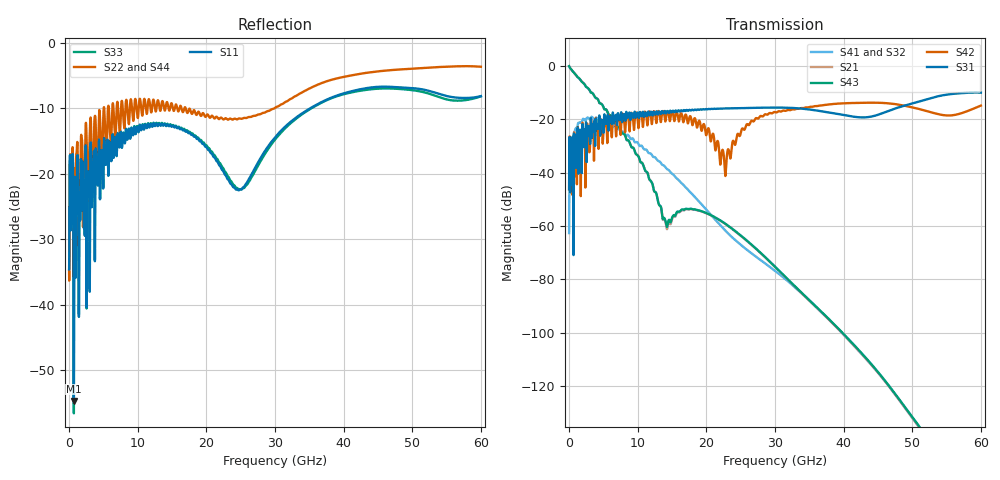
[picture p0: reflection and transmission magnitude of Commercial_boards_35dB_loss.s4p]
! Touchstone file from project Channel_builder
! Exported from Circuit Design 8.0.0
# GHZ S MA R 50.000000
! Modal data exported
! Port[1] = Port1
! Port[2] = Port2
! Port[3] = Port3
! Port[4] = Port4
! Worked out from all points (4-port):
!   12000 points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, 5 MHz to 60 GHz, reference 50 ohm
!   strongest paths, dB at 5 MHz, 15.01 GHz, 30 GHz, 45.01 GHz, 60 GHz:
!     S31: -46.3, -17.3, -15.7, -18.4, -10.1
!     S42: -46.3, -17.2, -17.4, -13.9, -14.9
!     S43: -0.2, -56.9, -75.3, -114.7, -182.1
!     S21: -0.2, -57.4, -75.4, -114.9, -183.0
!     S41: -62.7, -40.4, -76.8, -114.8, -182.6
!     S32: -62.7, -40.4, -76.8, -114.8, -182.3
!   lowest |S11| = -54.7 dB at 695 MHz (marker M1), VSWR 1.00, Z = 50.1 + j0.167 ohm
!   |S11| at or under -10 dB: start of sweep to 35.08 GHz
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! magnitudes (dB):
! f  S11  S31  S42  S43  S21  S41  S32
! 5 MHz  -34.6  -46.3  -46.3  -0.2  -0.2  -62.7  -62.7
! 695 MHz  -54.7  -28.4  -27.0  -2.5  -2.5  -25.2  -25.2
! 4.7 GHz  -17.0  -21.1  -23.8  -14.3  -14.3  -20.1  -20.1
! 14.22 GHz  -12.6  -17.4  -17.7  -60.2  -61.0  -38.6  -38.6
! 22.77 GHz  -20.2  -16.0  -41.3  -59.2  -59.2  -61.7  -61.8
! 31.59 GHz  -12.7  -15.7  -16.9  -79.3  -79.4  -80.1  -80.1
! 60 GHz  -8.1  -10.1  -14.9  -182.1  -183.0  -182.6  -182.3
